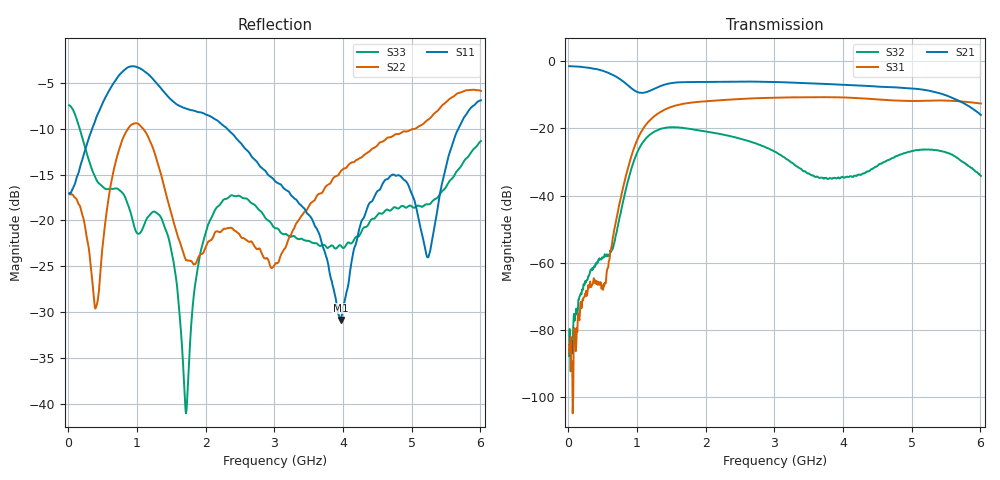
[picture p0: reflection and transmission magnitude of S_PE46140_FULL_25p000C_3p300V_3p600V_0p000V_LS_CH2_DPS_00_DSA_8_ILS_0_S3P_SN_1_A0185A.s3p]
! Device ID: PE46140_FULL
! File Path: z:\PE46140\MajorStates\25p000C\3p300\LS_CH2_DPS_00_DSA_8_ILS_0\PE46140_FULL_25p000C_3p300V_3p600V_0p000V_LS_CH2_DPS_00_DSA_8_ILS_0_S3P_SN_1_A0185A.s3p
! Serial: 1
! Lot: A0185A
! Temp: 25.000C
! VDD: 3.300
! VSS: 0.000
! Control_Hi: 3.600
! Control_Lo: 0.000
! Logic State: LS_CH2_DPS_00_DSA_8_ILS_0
! Port 1: RFIN
! Port 2: RFOUT1
! Port 3: RFOUT2
! ThroughPath:1-3
! IDD: 0.0003148247
! ISS: -1.769e-007
! Comment:
#  Hz  S  RI  R  50
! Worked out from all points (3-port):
!   801 points, 10 MHz to 6.01 GHz, reference 50 ohm
!   strongest paths, dB at 10 MHz, 1.51 GHz, 3.01 GHz, 4.51 GHz, 6.01 GHz:
!     S21: -1.5, -6.5, -6.2, -7.6, -16.0
!     S31: -85.9, -13.5, -10.9, -11.4, -12.6
!     S32: -87.8, -19.7, -27.0, -31.0, -34.2
!   lowest |S11| = -30.9 dB at 3.97 GHz (marker M1), VSWR 1.06, Z = 47.9 + j1.8 ohm
!   |S11| at or under -10 dB: start of sweep to 346.1 MHz; 2.31 GHz to 5.683 GHz (3.373 GHz wide, 84.4 % of centre)
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1e7  0.1401 -0.0109  0.842 -0.0245  -1.62e-06 4.48e-06
     0.8418 -0.0244  0.14 -0.00676  -5.84e-05 1.17e-05
     5e-05 8.97e-06  3.69e-05 1.75e-05  0.4226 -0.038
4.075e8  -0.0697 -0.3584  0.3635 -0.6664  -0.000434 -8.55e-05
         0.3648 -0.6703  -0.0311 -0.0145  2.16e-05 0.001
         -0.000479 -9.26e-06  5.51e-05 0.000942  -0.1639 -0.0299
1.1725e9  -0.5781 0.2285  -0.2079 -0.2897  -0.1266 -0.0107
          -0.2081 -0.2903  0.2053 -0.1892  0.00345 0.0782
          -0.1269 -0.011  0.00343 0.0781  0.0973 0.042
1.7125e9  -0.2765 0.2988  -0.4881 0.00692  0.1782 0.1535
          -0.4883 0.00686  0.0343 -0.0501  -0.0218 -0.0975
          0.1785 0.1538  -0.0218 -0.0976  0.00888 -3.12e-05
2.125e9  -0.1126 0.3401  -0.3398 0.3551  0.2189 -0.1365
         -0.34 0.355  0.0756 -0.0375  -0.0755 0.0399
         0.2192 -0.1367  -0.0754 0.0398  0.0928 0.0626
3.01e9  0.0415 0.1583  0.4049 0.2733  -0.2528 -0.1338
        0.4048 0.2742  -0.0575 -0.0019  0.0398 -0.0203
        -0.2533 -0.1339  0.0399 -0.0203  0.0908 -0.00184
3.97e9  -0.0216 0.0188  0.1022 -0.4346  -0.0294 0.2874
        0.1024 -0.4348  0.1296 0.1328  0.00991 0.0154
        -0.0293 0.2874  0.0102 0.0156  0.0721 0.0102
4.8025e9  -0.1759 -0.011  -0.4047 -0.0143  0.2562 0.0337
          -0.4049 -0.0151  0.294 0.0255  -0.0391 -0.00329
          0.2561 0.0332  -0.0392 -0.00306  0.1127 -0.0273
5.245e9  -0.0448 -0.0444  -0.1857 0.314  0.2086 -0.1518
         -0.1867 0.3135  0.3545 -0.016  -0.00478 0.0481
         0.2084 -0.1521  -0.0046 0.0482  0.1224 -0.0026
6.01e9  -0.3443 -0.2914  0.1512 0.0446  -0.1168 -0.202
        0.1516 0.0449  0.2474 -0.4433  0.0176 -0.00909
        -0.118 -0.2023  0.0173 -0.0091  0.2663 0.0479
